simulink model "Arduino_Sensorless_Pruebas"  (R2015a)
settings: Solver=ode45  StartTime=0.0  StopTime=10.0  RelTol=1e-3
libraries: dspsigops x12, arduinolib x11, simulink x6

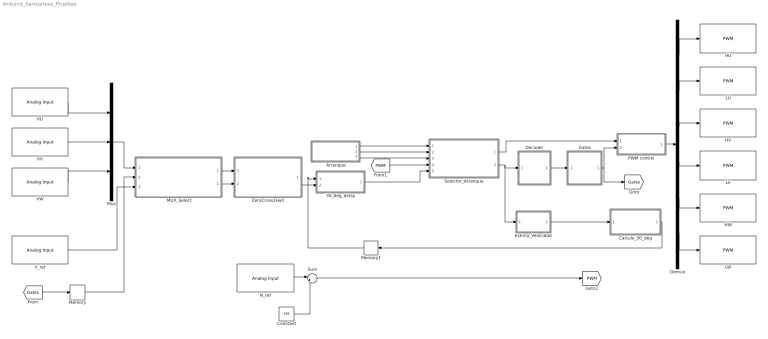
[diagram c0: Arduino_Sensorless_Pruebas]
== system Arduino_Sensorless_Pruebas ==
  " MUX_Select" : Subsystem
  30_deg_delay : Subsystem
  Arranque : Subsystem
  Calculo_30_deg : Subsystem
  Constant : Constant  Value=195
  Decoder : Subsystem
  Demux : Demux  Outputs=6
  Estima_Velocidad : Subsystem
  Gates : Subsystem
  HU : arduinolib/PWM  pinNumber=6  blockPlatform=arduino
  HV : arduinolib/PWM  pinNumber=4  blockPlatform=arduino
  HW : arduinolib/PWM  pinNumber=2  blockPlatform=arduino
  LU : arduinolib/PWM  pinNumber=7  blockPlatform=arduino
  LV : arduinolib/PWM  pinNumber=5  blockPlatform=arduino
  LW : arduinolib/PWM  pinNumber=3  blockPlatform=arduino
  Memory : Memory
  Memory1 : Memory
  Mux : Mux  Inputs=3
  N_ref : arduinolib/Analog Input  pinNumber=0  sampleTime=0.0001  blockPlatform=arduino
  PWM control : Subsystem
  Selector_Arranque : Subsystem
  Sum : Sum  Inputs=|++
  VU : arduinolib/Analog Input  pinNumber=1  sampleTime=0.0001  blockPlatform=arduino
  VV : arduinolib/Analog Input  pinNumber=2  sampleTime=0.0001  blockPlatform=arduino
  VW : arduinolib/Analog Input  pinNumber=3  sampleTime=0.0001  blockPlatform=arduino
  V_ref : arduinolib/Analog Input  pinNumber=4  sampleTime=0.0001  blockPlatform=arduino
  ZeroCross2Hall : Subsystem
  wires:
  VV/1 -> Mux/2
  VU/1 -> Mux/1
  VW/1 -> Mux/3
  Gates/1(Gates) -> [Gates], PWM control/2(Gates)
  Decoder/1(emf_abc) -> Gates/1("emf_abc ")
  PWM control/1(Pulsos) -> Demux/1
  Demux/1 -> HU/1
  Demux/2 -> LU/1
  Demux/3 -> HV/1
  Demux/4 -> LV/1
  Demux/5 -> HW/1
  Demux/6 -> LW/1
  [Gates] -> Memory/1
  Memory/1 -> " MUX_Select"/2(Gates)
  Mux/1 -> " MUX_Select"/1(Lectura_Fases)
  " MUX_Select"/1(Zero_Crossing) -> ZeroCross2Hall/1(zero_crossing)
  " MUX_Select"/2(Trigger) -> ZeroCross2Hall/2(trigger)
  ZeroCross2Hall/1(Hall) -> 30_deg_delay/2(Hall)
  Calculo_30_deg/1(Delay) -> Memory1/1
  Arranque/3(Hall_Arranque) -> Selector_Arranque/3(Hal_Arranque)
  Arranque/2(PWM_Arranque) -> Selector_Arranque/2(PWM_Arranque)
  Arranque/1(Trigger) -> Selector_Arranque/1(Trigger)
  Selector_Arranque/2(Hall) -> Estima_Velocidad/1(Hall), Decoder/1("Hall ")
  Selector_Arranque/1(PWM) -> PWM control/1(V control)
  30_deg_delay/1(Hall_Delay) -> Selector_Arranque/5(Hall_Regulacion)
  N_ref/1 -> Sum/1
  V_ref/1 -> " MUX_Select"/3("V_REF ")
  Memory1/1 -> 30_deg_delay/1(30_deg)
  Sum/1 -> [PWM]
  Estima_Velocidad/1(N_est) -> Calculo_30_deg/1(N_rpm)
  [PWM] -> Selector_Arranque/4(PWM_Regulacion)
  Constant/1 -> Sum/2

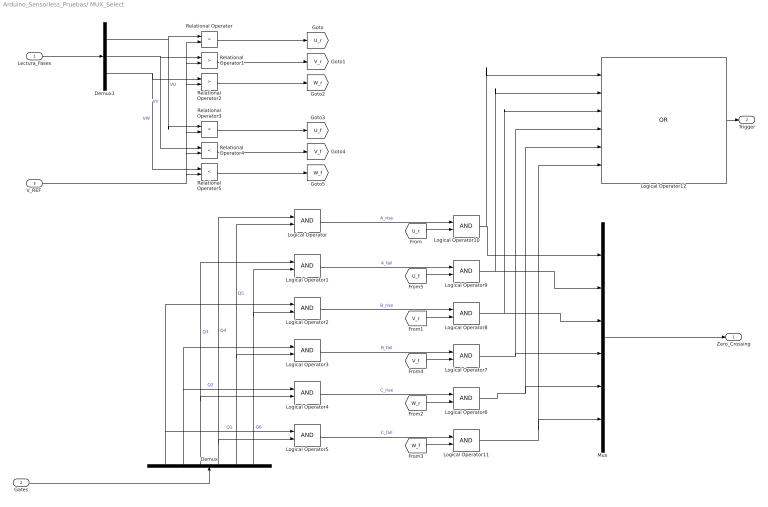
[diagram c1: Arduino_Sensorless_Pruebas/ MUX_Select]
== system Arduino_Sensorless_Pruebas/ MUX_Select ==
  Lectura_Fases : Inport
  Gates : Inport  Port=2
  "V_REF " : Inport  Port=3
  Demux : Demux  Outputs=6
  Demux1 : Demux  Outputs=3
  Logical Operator{,1..11} (12 alike) : Logic  IconShape=distinctive  AllPortsSameDT=off  OutDataTypeStr=boolean
  Logical Operator12 : Logic  Operator=OR  Inputs=6  AllPortsSameDT=off  OutDataTypeStr=boolean
  Mux : Mux  Inputs=6
  Relational Operator : RelationalOperator  Operator=>  OutDataTypeStr=boolean
  Relational Operator1 : RelationalOperator  Operator=>  OutDataTypeStr=boolean
  Relational Operator2 : RelationalOperator  Operator=>  OutDataTypeStr=boolean
  Relational Operator3 : RelationalOperator  Operator=<  OutDataTypeStr=boolean
  Relational Operator4 : RelationalOperator  Operator=<  OutDataTypeStr=boolean
  Relational Operator5 : RelationalOperator  Operator=<  OutDataTypeStr=boolean
  Zero_Crossing : Outport
  Trigger : Outport  Port=2
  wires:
  Gates/1 -> Demux/1
  Demux/1 -> Logical Operator5/1, Logical Operator2/1  "Q1"
  Demux/2 -> Logical Operator4/1, Logical Operator3/1  "Q2"
  Demux/3 -> Logical Operator4/2, Logical Operator1/1  "Q3"
  Demux/4 -> Logical Operator5/2, Logical Operator/1  "Q4"
  Demux/5 -> Logical Operator3/2, Logical Operator/2  "Q5"
  Demux/6 -> Logical Operator2/2, Logical Operator1/2  "Q6"
  Logical Operator2/1 -> Logical Operator8/1  "B_rise"
  Logical Operator3/1 -> Logical Operator7/1  "B_fall"
  Logical Operator/1 -> Logical Operator10/1  "A_rise"
  Logical Operator1/1 -> Logical Operator9/1  "A_fall"
  Logical Operator4/1 -> Logical Operator6/1  "C_rise"
  Logical Operator5/1 -> Logical Operator11/1  "C_fall"
  Relational Operator3/1 -> [U_f]
  Relational Operator4/1 -> [V_f]
  Relational Operator5/1 -> [W_f]
  [U_r] -> Logical Operator10/2
  [U_f] -> Logical Operator9/2
  [V_r] -> Logical Operator8/2
  [V_f] -> Logical Operator7/2
  [W_r] -> Logical Operator6/2
  [W_f] -> Logical Operator11/2
  Mux/1 -> Zero_Crossing/1
  Logical Operator6/1 -> Logical Operator12/5, Mux/5
  Logical Operator11/1 -> Mux/6, Logical Operator12/6
  Logical Operator7/1 -> Logical Operator12/4, Mux/4
  Logical Operator8/1 -> Logical Operator12/3, Mux/3
  Logical Operator9/1 -> Logical Operator12/2, Mux/2
  Logical Operator10/1 -> Logical Operator12/1, Mux/1
  Logical Operator12/1 -> Trigger/1
  Lectura_Fases/1 -> Demux1/1
  "V_REF "/1 -> Relational Operator4/2, Relational Operator3/2, Relational Operator2/2, Relational Operator1/2, Relational Operator/2, Relational Operator5/2
  Demux1/3 -> Relational Operator5/1, Relational Operator2/1  "VW"
  Demux1/1 -> Relational Operator3/1, Relational Operator/1  "VU"
  Demux1/2 -> Relational Operator4/1, Relational Operator1/1  "VV"
  Relational Operator2/1 -> [W_r]
  Relational Operator1/1 -> [V_r]
  Relational Operator/1 -> [U_r]

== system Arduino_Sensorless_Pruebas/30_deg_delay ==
  30_deg : Inport
  Hall : Inport  Port=2
  Data Type Conversion : DataTypeConversion  OutDataTypeStr=double
  Data Type Conversion1 : DataTypeConversion  OutDataTypeStr=boolean
  Variable Time Delay : VariableTransportDelay  MaximumDelay=10  MaximumPoints=256  FixedBuffer=on
  Hall_Delay : Outport
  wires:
  Hall/1 -> Data Type Conversion/1
  Data Type Conversion/1 -> Variable Time Delay/1
  30_deg/1 -> Variable Time Delay/2
  Variable Time Delay/1 -> Data Type Conversion1/1
  Data Type Conversion1/1 -> Hall_Delay/1

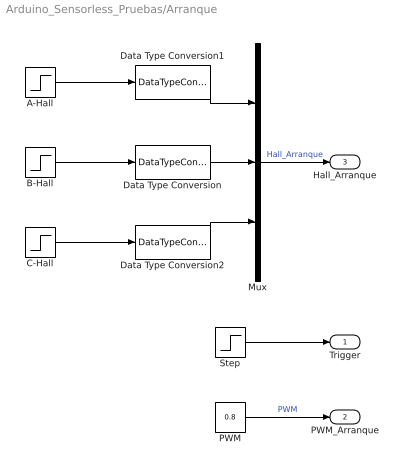
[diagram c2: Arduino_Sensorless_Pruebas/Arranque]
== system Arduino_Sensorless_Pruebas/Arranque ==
  A-Hall : Step  Time=8.364E-3  Before=1  After=0  SampleTime=0
  B-Hall : Step  Time=5.8145E-3  SampleTime=0
  C-Hall : Step  Time=10.8E-3  SampleTime=0
  Data Type Conversion : DataTypeConversion  OutDataTypeStr=boolean
  Data Type Conversion1 : DataTypeConversion  OutDataTypeStr=boolean
  Data Type Conversion2 : DataTypeConversion  OutDataTypeStr=boolean
  Mux : Mux  Inputs=3
  PWM : Constant  Value=0.8
  Step : Step  Time=13.25E-3  Before=0.5  After=-0.5  SampleTime=0
  Trigger : Outport
  PWM_Arranque : Outport  Port=2
  Hall_Arranque : Outport  Port=3
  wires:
  B-Hall/1 -> Data Type Conversion/1
  C-Hall/1 -> Data Type Conversion2/1
  A-Hall/1 -> Data Type Conversion1/1
  Data Type Conversion/1 -> Mux/2
  Data Type Conversion1/1 -> Mux/1
  Data Type Conversion2/1 -> Mux/3
  Mux/1 -> Hall_Arranque/1  "Hall_Arranque"
  Step/1 -> Trigger/1
  PWM/1 -> PWM_Arranque/1  "PWM"

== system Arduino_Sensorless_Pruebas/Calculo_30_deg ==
  N_rpm : Inport
  30_deg : Constant  Value=1/12
  Divide : Product  Inputs=*/
  Saturation : Saturate  UpperLimit=inf  LowerLimit=10
  Delay : Outport
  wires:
  30_deg/1 -> Divide/1
  Divide/1 -> Delay/1
  N_rpm/1 -> Saturation/1
  Saturation/1 -> Divide/2

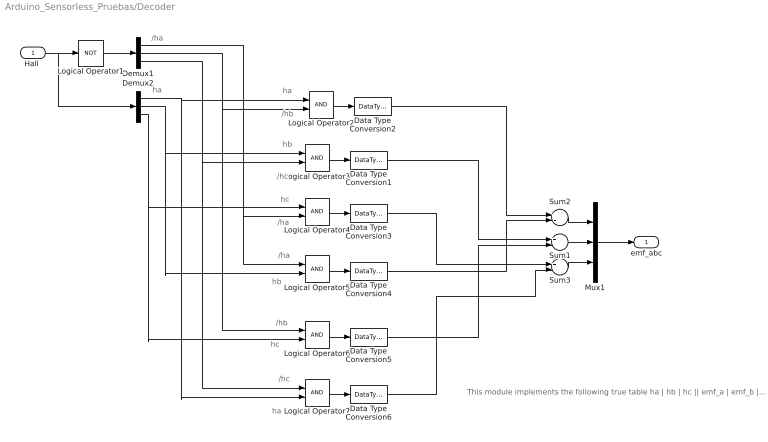
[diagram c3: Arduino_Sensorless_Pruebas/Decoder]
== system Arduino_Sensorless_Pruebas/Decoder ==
  note: /ha
  note: ha
  note: ha
  note: /hb
  note: hb
  note: /hc
  note: hc
  note: /ha
  note: /ha
  note: hb
  note: /hb
  note: hc
  note: /hc
  note: ha
  note: This module implements the following true table ha | hb | hc || emf_a | emf_b | emf_c -------------------------------------------------------------------------------- 0 0 0 0 0 0 0 0 1 0 -1 +1 0 1 0 -1 +1 0 0 1 1 -1 0 +1 1 0 0 +1 0 -1 1 0 1 +1 -1 0 1 1 0 0 +1 -1 1 1 1 0 0 0
  "Hall " : Inport
  Data Type Conversion{1..6} (6 alike) : DataTypeConversion
  Demux1 : Demux  Outputs=3
  Demux2 : Demux  Outputs=3
  Logical Operator1 : Logic  Operator=NOT  AllPortsSameDT=off  OutDataTypeStr=boolean
  Logical Operator{2..7} (6 alike) : Logic  AllPortsSameDT=off  OutDataTypeStr=boolean
  Mux1 : Mux  Inputs=3
  Sum1 : Sum  Inputs=+-  OutDataTypeStr=double
  Sum2 : Sum  Inputs=+-  OutDataTypeStr=double
  Sum3 : Sum  Inputs=+-  OutDataTypeStr=double
  emf_abc : Outport
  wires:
  "Hall "/1 -> Logical Operator1/1, Demux2/1
  Logical Operator1/1 -> Demux1/1
  Demux2/3 -> Logical Operator4/1, Logical Operator6/2
  Demux2/2 -> Logical Operator3/1, Logical Operator5/2
  Demux2/1 -> Logical Operator2/1, Logical Operator7/2
  Demux1/3 -> Logical Operator3/2, Logical Operator7/1
  Demux1/2 -> Logical Operator2/2, Logical Operator6/1
  Demux1/1 -> Logical Operator4/2, Logical Operator5/1
  Logical Operator2/1 -> Data Type Conversion2/1
  Sum2/1 -> Mux1/1
  Sum1/1 -> Mux1/2
  Sum3/1 -> Mux1/3
  Mux1/1 -> emf_abc/1
  Logical Operator3/1 -> Data Type Conversion1/1
  Logical Operator4/1 -> Data Type Conversion3/1
  Logical Operator5/1 -> Data Type Conversion4/1
  Logical Operator6/1 -> Data Type Conversion5/1
  Logical Operator7/1 -> Data Type Conversion6/1
  Data Type Conversion2/1 -> Sum2/1
  Data Type Conversion4/1 -> Sum2/2
  Data Type Conversion1/1 -> Sum1/1
  Data Type Conversion5/1 -> Sum1/2
  Data Type Conversion3/1 -> Sum3/1
  Data Type Conversion6/1 -> Sum3/2

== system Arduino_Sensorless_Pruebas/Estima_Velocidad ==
  Hall : Inport
  Demux : Demux  Outputs=3
  Estima_v_Fase_A : Subsystem
  Estima_v_Fase_B : Subsystem
  Estima_v_Fase_C : Subsystem
  Seleccion_estimada : Subsystem
  N_est : Outport
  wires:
  Demux/1 -> Estima_v_Fase_A/1(Hall_i)
  Hall/1 -> Seleccion_estimada/4(Hall), Demux/1
  Demux/3 -> Estima_v_Fase_C/1(Hall_i)
  Demux/2 -> Estima_v_Fase_B/1(Hall_i)
  Estima_v_Fase_A/1(Estimada_i) -> Seleccion_estimada/1(Estimada_A)
  Estima_v_Fase_B/1(Estimada_i) -> Seleccion_estimada/2(Estimada_B)
  Estima_v_Fase_C/1(Estimada_i) -> Seleccion_estimada/3(Estimada_C)
  Seleccion_estimada/1(Out1) -> N_est/1

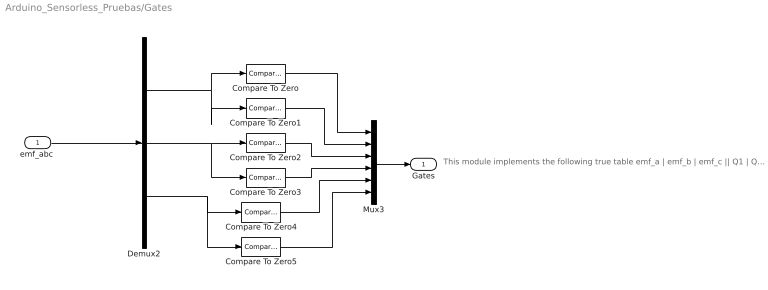
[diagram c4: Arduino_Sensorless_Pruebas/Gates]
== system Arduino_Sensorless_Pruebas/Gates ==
  note: This module implements the following true table emf_a | emf_b | emf_c || Q1 | Q2 | Q3 | Q4 | Q5 | Q6 ------------------------------------------------------------------------------------------------------------------ 0 0 0 0 0 0 0 0 0 0 -1 +1 0 0 0 1 1 0 -1 +1 0 0 1 1 0 0 0 -1 0 +1 0 1 0 0 1 0 +1 0 -1 1 0 0 0 0 1 +1 -1 0 1 0 0 1 0 0 0 +1 -1 0 0 1 0 0 1 0 0 0 0 0 0 0 0 0
  "emf_abc " : Inport
  Compare To Zero : simulink/Logic and Bit Operations/Compare To Zero  relop=>  OutDataTypeStr=boolean  ZeroCross=off
  Compare To Zero1 : simulink/Logic and Bit Operations/Compare To Zero  relop=<  OutDataTypeStr=boolean  ZeroCross=off
  Compare To Zero2 : simulink/Logic and Bit Operations/Compare To Zero  relop=>  OutDataTypeStr=boolean  ZeroCross=off
  Compare To Zero3 : simulink/Logic and Bit Operations/Compare To Zero  relop=<  OutDataTypeStr=boolean  ZeroCross=off
  Compare To Zero4 : simulink/Logic and Bit Operations/Compare To Zero  relop=>  OutDataTypeStr=boolean  ZeroCross=off
  Compare To Zero5 : simulink/Logic and Bit Operations/Compare To Zero  relop=<  OutDataTypeStr=boolean  ZeroCross=off
  Demux2 : Demux  Outputs=3
  Mux3 : Mux  Inputs=6
  Gates : Outport
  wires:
  "emf_abc "/1 -> Demux2/1
  Mux3/1 -> Gates/1
  Demux2/1 -> Compare To Zero/1, Compare To Zero1/1
  Demux2/2 -> Compare To Zero2/1, Compare To Zero3/1
  Demux2/3 -> Compare To Zero4/1, Compare To Zero5/1
  Compare To Zero/1 -> Mux3/1
  Compare To Zero1/1 -> Mux3/2
  Compare To Zero2/1 -> Mux3/3
  Compare To Zero3/1 -> Mux3/4
  Compare To Zero4/1 -> Mux3/5
  Compare To Zero5/1 -> Mux3/6

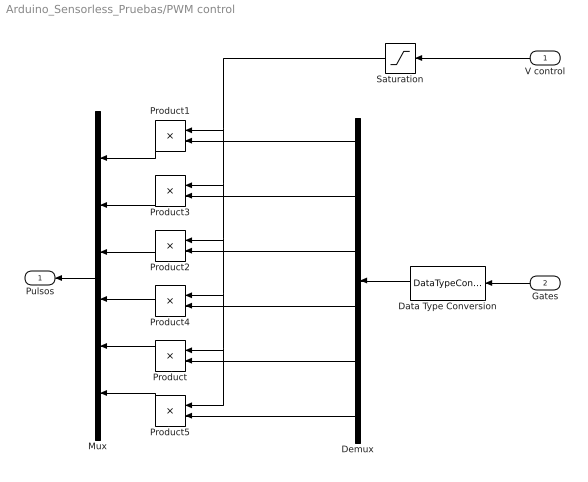
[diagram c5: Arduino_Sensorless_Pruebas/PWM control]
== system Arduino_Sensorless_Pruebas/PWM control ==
  V control : Inport
  Gates : Inport  Port=2
  Data Type Conversion : DataTypeConversion  OutDataTypeStr=double
  Demux : Demux  Outputs=6
  Mux : Mux  Inputs=6
  Product{,1..5} (6 alike) : Product
  Saturation : Saturate  UpperLimit=255  LowerLimit=0
  Pulsos : Outport
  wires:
  Gates/1 -> Data Type Conversion/1
  Data Type Conversion/1 -> Demux/1
  Mux/1 -> Pulsos/1
  Product1/1 -> Mux/1
  Product2/1 -> Mux/3
  Product/1 -> Mux/5
  Demux/5 -> Product/2
  Demux/3 -> Product2/2
  Demux/1 -> Product1/2
  V control/1 -> Saturation/1
  Product5/1 -> Mux/6
  Demux/6 -> Product5/2
  Product4/1 -> Mux/4
  Demux/4 -> Product4/2
  Product3/1 -> Mux/2
  Demux/2 -> Product3/2
  Saturation/1 -> Product3/1, Product4/1, Product/1, Product5/1, Product2/1, Product1/1

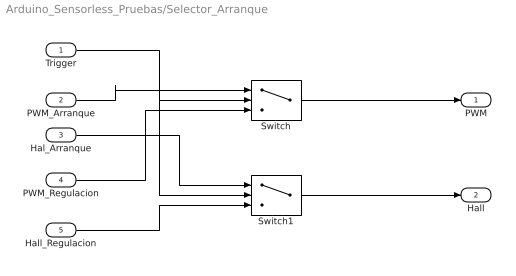
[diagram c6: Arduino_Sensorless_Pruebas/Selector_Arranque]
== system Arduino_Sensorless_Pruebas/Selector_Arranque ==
  Trigger : Inport
  PWM_Arranque : Inport  Port=2
  Hal_Arranque : Inport  Port=3
  PWM_Regulacion : Inport  Port=4
  Hall_Regulacion : Inport  Port=5
  Switch : Switch  Criteria=u2 > Threshold
  Switch1 : Switch  Criteria=u2 > Threshold
  PWM : Outport
  Hall : Outport  Port=2
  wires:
  Trigger/1 -> Switch1/2, Switch/2
  Hall_Regulacion/1 -> Switch1/3
  PWM_Regulacion/1 -> Switch/3
  Hal_Arranque/1 -> Switch1/1
  PWM_Arranque/1 -> Switch/1
  Switch/1 -> PWM/1
  Switch1/1 -> Hall/1

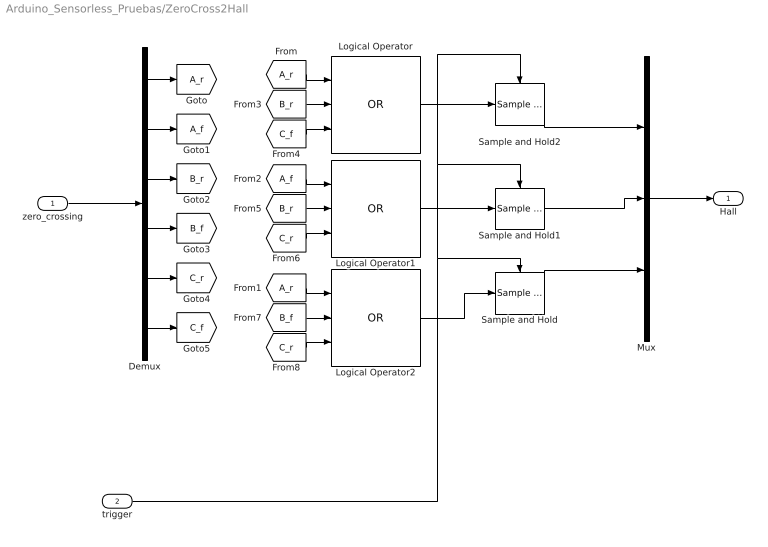
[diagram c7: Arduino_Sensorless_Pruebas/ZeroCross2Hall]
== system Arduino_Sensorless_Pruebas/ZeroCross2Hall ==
  zero_crossing : Inport
  trigger : Inport  Port=2
  Demux : Demux  Outputs=6
  Logical Operator : Logic  Operator=OR  Inputs=3  IconShape=distinctive  AllPortsSameDT=off  OutDataTypeStr=boolean
  Logical Operator1 : Logic  Operator=OR  Inputs=3  IconShape=distinctive  AllPortsSameDT=off  OutDataTypeStr=boolean
  Logical Operator2 : Logic  Operator=OR  Inputs=3  IconShape=distinctive  AllPortsSameDT=off  OutDataTypeStr=boolean
  Mux : Mux  Inputs=3
  Sample and Hold : dspsigops/Sample and Hold  trig=Rising edge  initCond=0  latchinput=off
  Sample and Hold1 : dspsigops/Sample and Hold  trig=Rising edge  initCond=0  latchinput=off
  Sample and Hold2 : dspsigops/Sample and Hold  trig=Rising edge  initCond=0  latchinput=off
  Hall : Outport
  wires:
  zero_crossing/1 -> Demux/1
  Mux/1 -> Hall/1
  trigger/1 -> Sample and Hold/Trigger, Sample and Hold1/Trigger, Sample and Hold2/Trigger
  Logical Operator2/1 -> Sample and Hold/1
  Sample and Hold/1 -> Mux/3
  Sample and Hold1/1 -> Mux/2
  Sample and Hold2/1 -> Mux/1
  Logical Operator1/1 -> Sample and Hold1/1
  Logical Operator/1 -> Sample and Hold2/1
  Demux/1 -> [A_r]
  Demux/6 -> [C_f]
  Demux/3 -> [B_r]
  Demux/2 -> [A_f]
  Demux/4 -> [B_f]
  Demux/5 -> [C_r]
  [A_r] -> Logical Operator2/1
  [A_r] -> Logical Operator/1
  [A_f] -> Logical Operator1/1
  [B_r] -> Logical Operator/2
  [C_f] -> Logical Operator/3
  [B_r] -> Logical Operator1/2
  [C_r] -> Logical Operator1/3
  [C_r] -> Logical Operator2/3
  [B_f] -> Logical Operator2/2

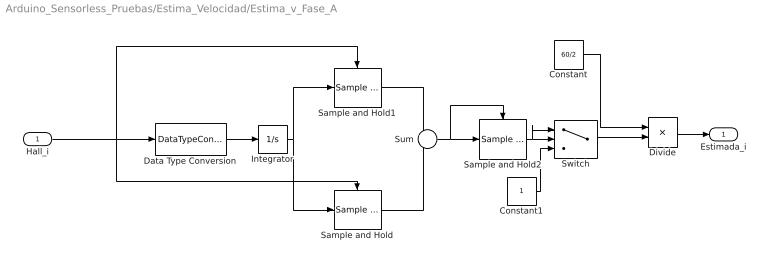
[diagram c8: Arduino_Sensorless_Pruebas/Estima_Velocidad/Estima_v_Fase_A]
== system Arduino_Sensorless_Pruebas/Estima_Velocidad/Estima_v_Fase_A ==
  Hall_i : Inport
  Constant : Constant  Value=60/2
  Constant1 : Constant
  Data Type Conversion : DataTypeConversion  OutDataTypeStr=double
  Divide : Product  Inputs=*/
  Integrator : Integrator
  Sample and Hold : dspsigops/Sample and Hold  trig=Rising edge  initCond=0  latchinput=off
  Sample and Hold1 : dspsigops/Sample and Hold  trig=Falling edge  initCond=0  latchinput=off
  Sample and Hold2 : dspsigops/Sample and Hold  trig=Rising edge  initCond=0  latchinput=off
  Sum : Sum  Inputs=+|-
  Switch : Switch  Criteria=u2 > Threshold
  Estimada_i : Outport
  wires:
  Hall_i/1 -> Data Type Conversion/1, Sample and Hold/Trigger, Sample and Hold1/Trigger
  Integrator/1 -> Sample and Hold1/1, Sample and Hold/1
  Sample and Hold/1 -> Sum/2
  Sample and Hold1/1 -> Sum/1
  Sum/1 -> Sample and Hold2/Trigger, Sample and Hold2/1
  Sample and Hold2/1 -> Switch/1, Switch/2
  Constant/1 -> Divide/1
  Switch/1 -> Divide/2
  Constant1/1 -> Switch/3
  Divide/1 -> Estimada_i/1
  Data Type Conversion/1 -> Integrator/1

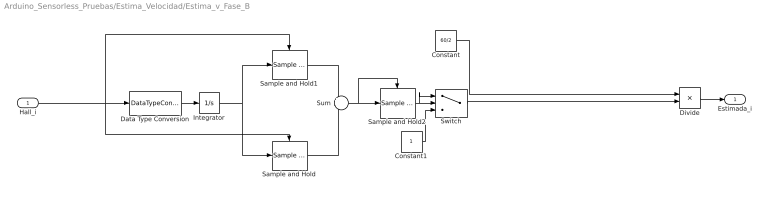
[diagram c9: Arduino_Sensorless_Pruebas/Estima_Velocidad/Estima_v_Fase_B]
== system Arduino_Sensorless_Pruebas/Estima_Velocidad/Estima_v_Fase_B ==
  Hall_i : Inport
  Constant : Constant  Value=60/2
  Constant1 : Constant
  Data Type Conversion : DataTypeConversion  OutDataTypeStr=double
  Divide : Product  Inputs=*/
  Integrator : Integrator
  Sample and Hold : dspsigops/Sample and Hold  trig=Rising edge  initCond=0  latchinput=off
  Sample and Hold1 : dspsigops/Sample and Hold  trig=Falling edge  initCond=0  latchinput=off
  Sample and Hold2 : dspsigops/Sample and Hold  trig=Rising edge  initCond=0  latchinput=off
  Sum : Sum  Inputs=+|-
  Switch : Switch  Criteria=u2 > Threshold
  Estimada_i : Outport
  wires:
  Hall_i/1 -> Data Type Conversion/1, Sample and Hold/Trigger, Sample and Hold1/Trigger
  Integrator/1 -> Sample and Hold1/1, Sample and Hold/1
  Sample and Hold/1 -> Sum/2
  Sample and Hold1/1 -> Sum/1
  Sum/1 -> Sample and Hold2/Trigger, Sample and Hold2/1
  Sample and Hold2/1 -> Switch/1, Switch/2
  Constant/1 -> Divide/1
  Switch/1 -> Divide/2
  Constant1/1 -> Switch/3
  Divide/1 -> Estimada_i/1
  Data Type Conversion/1 -> Integrator/1

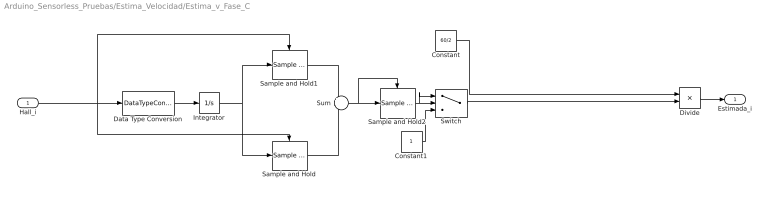
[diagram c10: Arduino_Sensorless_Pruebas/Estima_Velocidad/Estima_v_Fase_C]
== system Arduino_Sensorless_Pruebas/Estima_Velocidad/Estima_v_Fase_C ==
  Hall_i : Inport
  Constant : Constant  Value=60/2
  Constant1 : Constant
  Data Type Conversion : DataTypeConversion  OutDataTypeStr=double
  Divide : Product  Inputs=*/
  Integrator : Integrator
  Sample and Hold : dspsigops/Sample and Hold  trig=Rising edge  initCond=0  latchinput=off
  Sample and Hold1 : dspsigops/Sample and Hold  trig=Falling edge  initCond=0  latchinput=off
  Sample and Hold2 : dspsigops/Sample and Hold  trig=Rising edge  initCond=0  latchinput=off
  Sum : Sum  Inputs=+|-
  Switch : Switch  Criteria=u2 > Threshold  Threshold=3E-5
  Estimada_i : Outport
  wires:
  Hall_i/1 -> Data Type Conversion/1, Sample and Hold/Trigger, Sample and Hold1/Trigger
  Integrator/1 -> Sample and Hold1/1, Sample and Hold/1
  Sample and Hold/1 -> Sum/2
  Sample and Hold1/1 -> Sum/1
  Sum/1 -> Sample and Hold2/Trigger, Sample and Hold2/1
  Sample and Hold2/1 -> Switch/1, Switch/2
  Constant/1 -> Divide/1
  Switch/1 -> Divide/2
  Constant1/1 -> Switch/3
  Divide/1 -> Estimada_i/1
  Data Type Conversion/1 -> Integrator/1

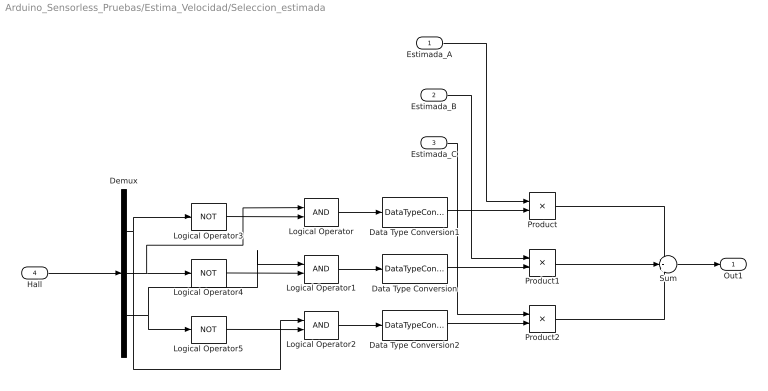
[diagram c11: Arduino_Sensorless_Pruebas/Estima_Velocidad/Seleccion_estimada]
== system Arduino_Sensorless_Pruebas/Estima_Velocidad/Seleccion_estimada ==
  Estimada_A : Inport
  Estimada_B : Inport  Port=2
  Estimada_C : Inport  Port=3
  Hall : Inport  Port=4
  Data Type Conversion : DataTypeConversion  OutDataTypeStr=double
  Data Type Conversion1 : DataTypeConversion  OutDataTypeStr=double
  Data Type Conversion2 : DataTypeConversion  OutDataTypeStr=double
  Demux : Demux  Outputs=3
  Logical Operator : Logic  IconShape=distinctive  AllPortsSameDT=off  OutDataTypeStr=boolean
  Logical Operator1 : Logic  IconShape=distinctive  AllPortsSameDT=off  OutDataTypeStr=boolean
  Logical Operator2 : Logic  IconShape=distinctive  AllPortsSameDT=off  OutDataTypeStr=boolean
  Logical Operator3 : Logic  Operator=NOT  IconShape=distinctive  AllPortsSameDT=off  OutDataTypeStr=boolean
  Logical Operator4 : Logic  Operator=NOT  IconShape=distinctive  AllPortsSameDT=off  OutDataTypeStr=boolean
  Logical Operator5 : Logic  Operator=NOT  IconShape=distinctive  AllPortsSameDT=off  OutDataTypeStr=boolean
  Product : Product
  Product1 : Product
  Product2 : Product
  Sum : Sum  Inputs=+++
  Out1 : Outport
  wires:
  Hall/1 -> Demux/1
  Product/1 -> Sum/1
  Product1/1 -> Sum/2
  Product2/1 -> Sum/3
  Logical Operator3/1 -> Logical Operator/2
  Logical Operator4/1 -> Logical Operator1/2
  Logical Operator5/1 -> Logical Operator2/2
  Demux/3 -> Logical Operator1/1, Logical Operator5/1
  Demux/2 -> Logical Operator/1, Logical Operator4/1
  Demux/1 -> Logical Operator2/1, Logical Operator3/1
  Logical Operator1/1 -> Data Type Conversion/1
  Logical Operator2/1 -> Data Type Conversion2/1
  Logical Operator/1 -> Data Type Conversion1/1
  Sum/1 -> Out1/1
  Estimada_C/1 -> Product2/1
  Data Type Conversion2/1 -> Product2/2
  Data Type Conversion/1 -> Product1/2
  Data Type Conversion1/1 -> Product/2
  Estimada_B/1 -> Product1/1
  Estimada_A/1 -> Product/1
